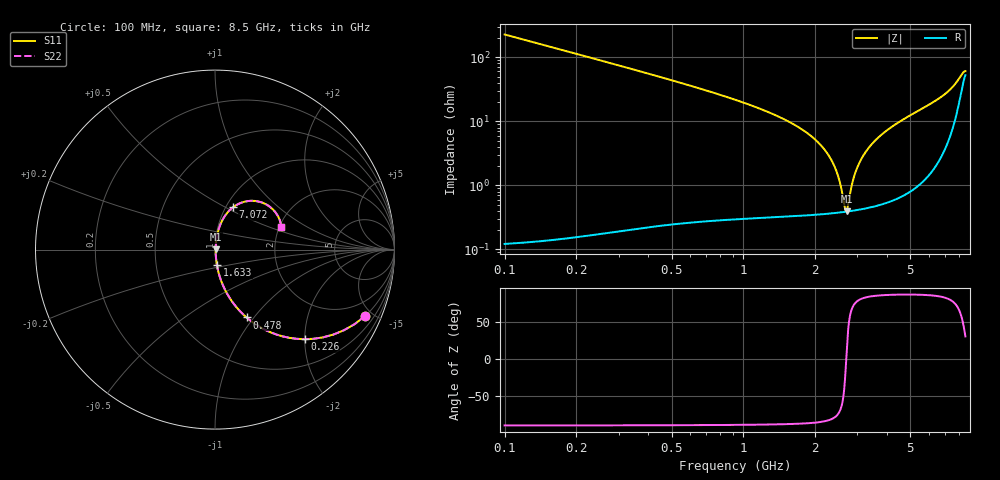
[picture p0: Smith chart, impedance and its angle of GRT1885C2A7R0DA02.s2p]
!Murata Part Number: GRT1885C2A7R0DA02
!These Parameters are Measured in Series Mode Connection
!Data Generated on Jun 19, 2026
!  o--ll--o
!Port1  Port2
!  o------o
!Operation Temp=25[degC], DC Bias Voltage=0[V]
!Freq. Start=100[MHz] Stop=9[GHz] 401[Steps]
# Hz S RI R 50
!Freq.(Hz) S11(Real) S11(Imag) S21(Real) S21(Imag) S12(Real) S12(Imag) S22(Real) S22(Imag)
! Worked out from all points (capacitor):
!   401 points, 100 MHz to 8.5 GHz, reference 50 ohm
!   read as one part in series: C = 7 pF near 142 MHz
!   lowest |Z| = 394 mohm at 2.704 GHz (marker M1)
!   series resonance near 2.694 GHz, so ESL is about 500 pH
!   S11 on the Smith chart (normalised r, x): 100 MHz: 1.00, -4.54; 226 MHz: 1.00, -2.00; 478 MHz: 1.00, -0.92; 1.633 GHz: 1.01, -0.18; 7.072 GHz: 1.08, +0.55; 8.5 GHz: 2.05, +0.61
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1e8  0.8373 -0.3688  0.1627 0.3688  0.1627 0.3688  0.8373 -0.3688
2.26e8  0.4991 -0.4992  0.5009 0.4992  0.5009 0.4992  0.4991 -0.4992
3.31e8  0.314 -0.4626  0.686 0.4626  0.686 0.4626  0.314 -0.4626
4.78e8  0.176 -0.3782  0.824 0.3782  0.824 0.3782  0.176 -0.3782
8.35e8  0.0595 -0.2307  0.9405 0.2307  0.9405 0.2307  0.0595 -0.2307
1.507e9  0.0139 -0.1024  0.9861 0.1024  0.9861 0.1024  0.0139 -0.1024
1.633e9  0.011 -0.0873  0.989 0.0873  0.989 0.0873  0.011 -0.0873
2.053e9  0.00567 -0.0465  0.9943 0.0465  0.9943 0.0465  0.00567 -0.0465
2.326e9  0.00427 -0.0251  0.9957 0.0251  0.9957 0.0251  0.00427 -0.0251
2.494e9  0.00391 -0.0132  0.9961 0.0132  0.9961 0.0132  0.00391 -0.0132
2.662e9  0.00385 -0.00206  0.9961 0.00206  0.9961 0.00206  0.00385 -0.00206
2.704e9  0.00388 0.00062  0.9961 -0.00062  0.9961 -0.00062  0.00388 0.00062
2.914e9  0.00422 0.0135  0.9958 -0.0135  0.9958 -0.0135  0.00422 0.0135
3.103e9  0.00481 0.0245  0.9952 -0.0245  0.9952 -0.0245  0.00481 0.0245
3.397e9  0.00617 0.0406  0.9938 -0.0406  0.9938 -0.0406  0.00617 0.0406
3.775e9  0.00865 0.0603  0.9913 -0.0603  0.9913 -0.0603  0.00865 0.0603
4.3e9  0.0135 0.0863  0.9865 -0.0863  0.9865 -0.0863  0.0135 0.0863
5.707e9  0.0371 0.1561  0.9629 -0.1561  0.9629 -0.1561  0.0371 0.1561
7.072e9  0.1017 0.2368  0.8983 -0.2368  0.8983 -0.2368  0.1017 0.2368
7.114e9  0.1055 0.2396  0.8945 -0.2396  0.8945 -0.2396  0.1055 0.2396
7.975e9  0.2497 0.266  0.7503 -0.266  0.7503 -0.266  0.2497 0.266
8.5e9  0.3698 0.1255  0.6302 -0.1255  0.6302 -0.1255  0.3698 0.1255
